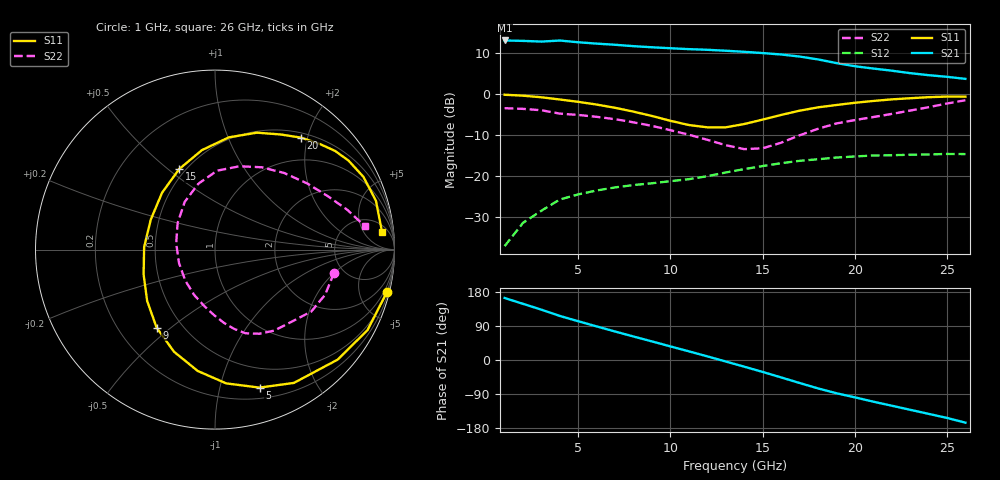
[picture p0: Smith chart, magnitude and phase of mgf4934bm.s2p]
! MGF4934BM  (VDS=2V, lDS=10mA, Ta=room temperature)
! S-parameters f=1-26GHz
! Board: er=2.6, 0.36mmt.
! 19/Sept./2007
# GHz S MA R 50
!  f  S11  S21  S12  S22
! (GHz)  Magn.  Angle  Magn.  Angle  Magn.  Angle  Magn.  Angle
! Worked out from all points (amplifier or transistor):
!   26 points, 1 GHz to 26 GHz, reference 50 ohm
!   highest |S21| = 13.1 dB at 1 GHz (marker M1)
!   |S21| within 3 dB of that: start of sweep to 14.76 GHz
!   unconditionally stable (mu >= 1): 8.431 GHz to 14.8 GHz
!   at 5 GHz: K = 0.58, MSG = 18.6 dB, |S12| = -24.4 dB
!   at 14 GHz: K = 1.07, MAG = 12.6 dB, |S12| = -18.3 dB
!   at 26 GHz: K = 0.26, MSG = 9.2 dB, |S12| = -14.6 dB
!   lowest NFmin = 0.25 dB at 1 GHz
!   S11 on the Smith chart (normalised r, x): 1 GHz: 0.47, -8.12; 5 GHz: 0.30, -1.33; 9 GHz: 0.36, -0.45; 15 GHz: 0.46, +0.55; 20 GHz: 0.58, +1.89; 26 GHz: 9, +14
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1  0.986 -14.0  4.534 163.6  0.014 79.1  0.676 -11.0
2  0.961 -27.8  4.478 148.2  0.027 70.5  0.663 -22.3
3  0.918 -41.9  4.394 132.8  0.038 61.9  0.638 -32.7
4  0.863 -59.4  4.523 116.2  0.052 50.3  0.58 -45.1
5  0.808 -72.1  4.309 102.2  0.06 43.3  0.559 -53.8
6  0.748 -85.2  4.148 88.6  0.067 36.9  0.53 -62.2
7  0.683 -98.1  4.015 75.1  0.073 30.5  0.496 -70.0
9  0.543 -126.8  3.744 49.0  0.082 20.9  0.411 -83.1
10  0.474 -142.9  3.644 35.8  0.087 17.1  0.364 -91.0
11  0.421 -160.9  3.552 22.8  0.092 14.0  0.321 -100.6
12  0.395 177.9  3.488 9.6  0.1 11.1  0.278 -114.7
13  0.395 154.9  3.396 -4.0  0.111 7.6  0.239 -133.9
14  0.433 132.9  3.295 -17.6  0.122 2.2  0.214 -159.5
15  0.491 114.0  3.183 -31.5  0.133 -4.2  0.219 170.8
16  0.559 97.5  3.056 -45.9  0.144 -11.1  0.256 144.4
17  0.63 83.0  2.886 -60.6  0.154 -18.6  0.315 122.4
18  0.692 70.3  2.662 -74.9  0.161 -26.6  0.379 104.1
19  0.739 60.2  2.401 -87.7  0.169 -34.2  0.44 88.4
20  0.787 52.4  2.198 -98.5  0.174 -42.1  0.484 73.6
22  0.866 39.4  1.94 -120.6  0.18 -58.5  0.575 47.9
24  0.921 26.1  1.71 -142.1  0.184 -71.5  0.695 25.4
26  0.936 5.9  1.541 -165.3  0.186 -86.0  0.846 8.8
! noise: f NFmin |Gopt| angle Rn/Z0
1  0.25  0.99  7.2  0.34
2  0.26  0.98  11.1  0.31
3  0.27  0.95  18  0.27
5  0.31  0.89  38.5  0.21
6  0.33  0.82  53.1  0.18
8  0.38  0.67  83.3  0.12
9  0.41  0.6  100.2  0.09
11  0.48  0.47  131.4  0.04
12  0.51  0.42  150.3  0.03
14  0.58  0.35  -178.8  0.03
